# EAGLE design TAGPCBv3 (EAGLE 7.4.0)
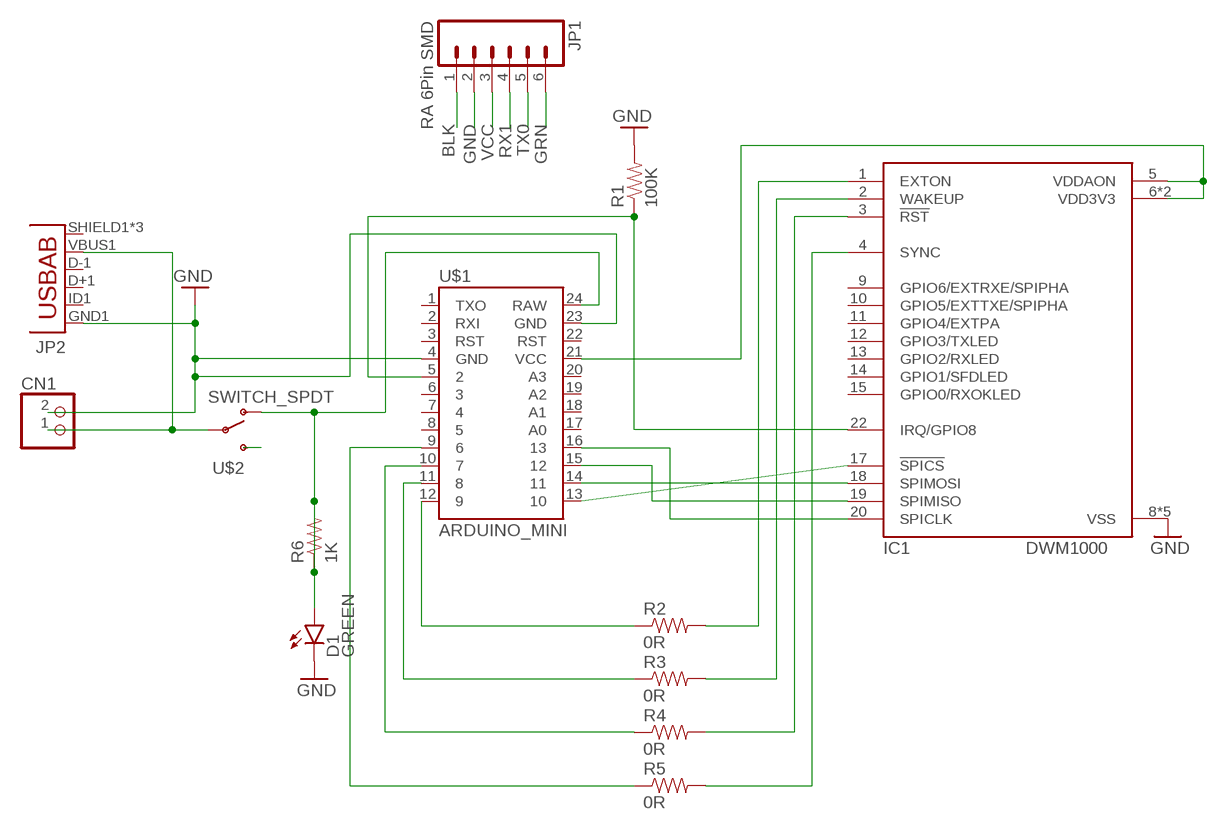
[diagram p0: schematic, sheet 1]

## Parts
CN1  JST_2PIN-SMT-RA  [JST-PH-2-SMT-RA]
D1  GREEN  LED-GREEN0603  [LED-0603]
IC1  DWM1000  [DWM1000]
JP1  RA 6Pin SMD  M06SMD  [1X06-SMD]
JP2  USB-ABCONN-11794  [USB-AB-MICRO-SMD_V03]
R1  100K  RESISTORAXIAL-0.3  [AXIAL-0.3]
R2  0R  RESISTOR1206  [1206]
R3  0R  RESISTOR1206  [1206]
R4  0R  RESISTOR1206  [1206]
R5  0R  RESISTOR1206  [1206]
R6  1K  RESISTOR1206  [1206]
U$1  ARDUINO_MINI  [ARDUINO_MINI]
U$2  SWITCH_SPDT  [KPS-1290]

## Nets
BLK: JP1.1
GND: CN1.2 D1.C IC1.8(VSS) IC1.16(VSS) IC1.21(VSS) IC1.23(VSS) IC1.24(VSS) JP1.2 JP2.GND1(GND) R1.P$2 U$1.4(GND) U$1.23(GND)
GRN: JP1.6
N$1: IC1.17(!SPICS) U$1.13
N$2: IC1.22(IRQ/GPIO8) R1.P$1 U$1.5
N$3: IC1.18(SPIMOSI) U$1.14
N$4: IC1.19(SPIMISO) U$1.15
N$5: IC1.20(SPICLK) U$1.16
N$6: D1.A R6.1 R6.2 U$1.24(RAW) U$2.O
N$7: CN1.1 JP2.VBUS1(VBUS) U$2.P
N$8: IC1.5(VDDAON) IC1.6(VDD3V3) IC1.7(VDD3V3) U$1.21(VCC)
N$9: R2.1 U$1.12
N$10: IC1.1(EXTON) R2.2
N$11: R3.1 U$1.11
N$12: IC1.2(WAKEUP) R3.2
N$13: IC1.3(!RST) R4.2
N$14: R4.1 U$1.10
N$15: R5.1 U$1.9
N$16: IC1.4(SYNC) R5.2
N$17: U$2.S
RX1: JP1.4
TX0: JP1.5
VCC: JP1.3
Unconnected: IC1.9(GPIO6/EXTRXE/SPIPHA) IC1.10(GPIO5/EXTTXE/SPIPHA) IC1.11(GPIO4/EXTPA) IC1.12(GPIO3/TXLED) IC1.13(GPIO2/RXLED) IC1.14(GPIO1/SFDLED) IC1.15(GPIO0/RXOKLED) JP2.D+1(D+) JP2.D-1(D-) JP2.ID1(USBID) JP2.SHIELD1(SHIELD) JP2.SHIELD2(SHIELD) JP2.SHIELD3(SHIELD) U$1.1(TXO) U$1.2(RXI) U$1.3(RST) U$1.6 U$1.7 U$1.8 U$1.17(A0) U$1.18(A1) U$1.19(A2) U$1.20(A3) U$1.22(RST)

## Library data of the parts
CN1 = adafruit:JST_2PIN: JST 2-Pin Connectors of various flavors
D1 = SparkFun-LED:LED-GREEN: Various green LEDs; PROD_ID: DIO-00821
IC1 = decawave:DWM1000
JP1 = SparkFun-Connectors:M06: Header 6 Standard 6-pin 0.1" header. Use with straight break away headers (SKU : PRT-00116), right angle break away headers (PRT-00553), swiss pins (PRT-00743), machine pins (PRT-00117), and female headers (PRT-00115). Molex polarized connector foot print use with SKU : PRT-08094 with associated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; PROD_ID: CONN-08971
JP2 = SparkFun-Connectors:USB-AB: This is a USB AB connector that is compatible with USB OTG. i.e. this connector can serve as a host or device; PROD_ID: CONN-11794
R1-R6 = SparkFun-Resistors:RESISTOR: Resistor
U$1 = SparkFun-Boards:ARDUINO_MINI: Arduino Pro Mini footprint
U$2 = SparkFun-Electromechanical:SWITCH_SPDT: SWCH-10651 Side-actuated SPDT slide switch, as used on the Arduino Pro; PROD_ID: SWCH-10651

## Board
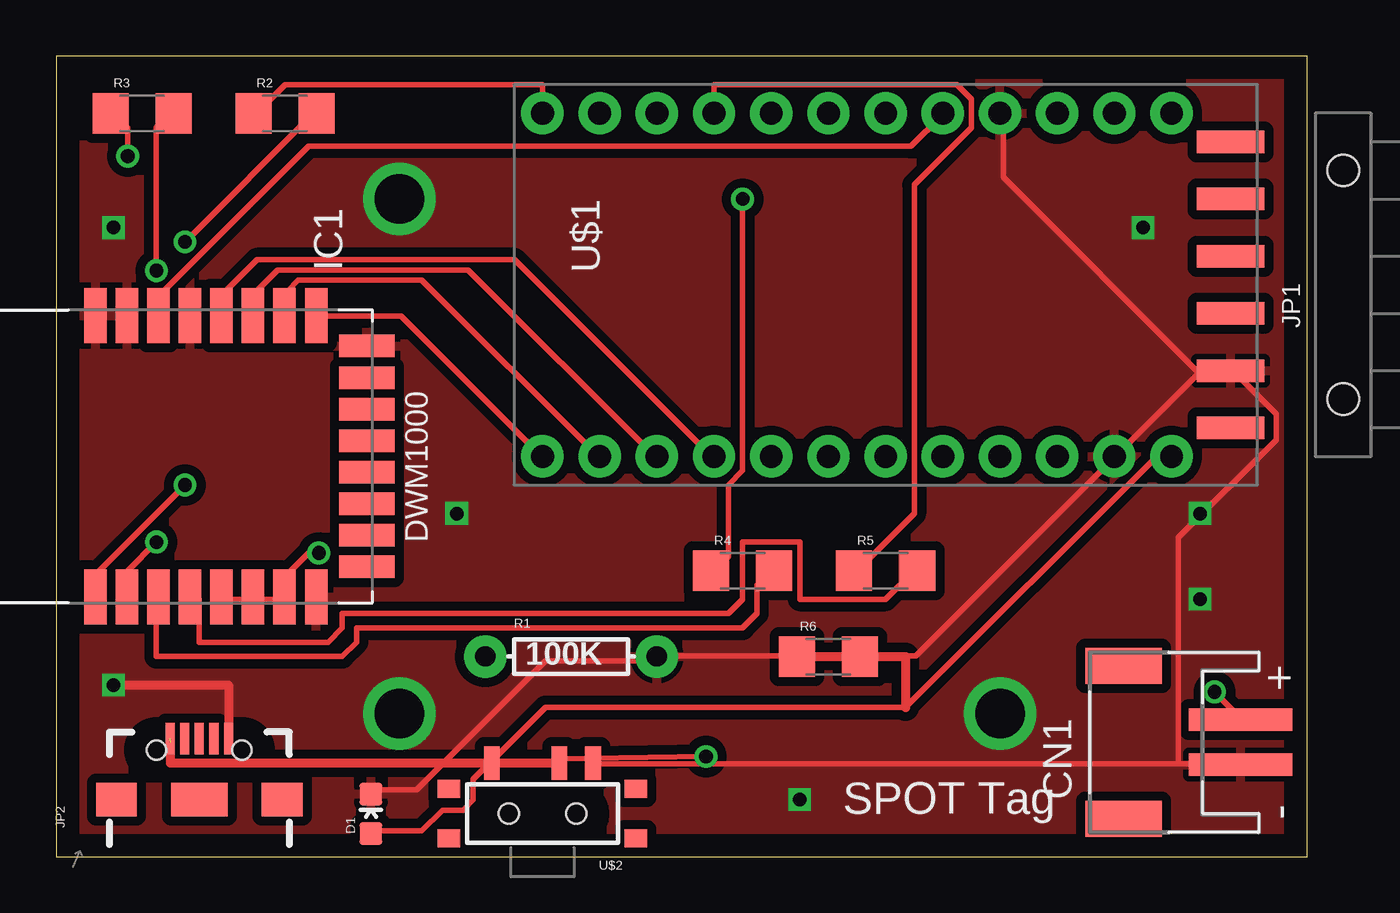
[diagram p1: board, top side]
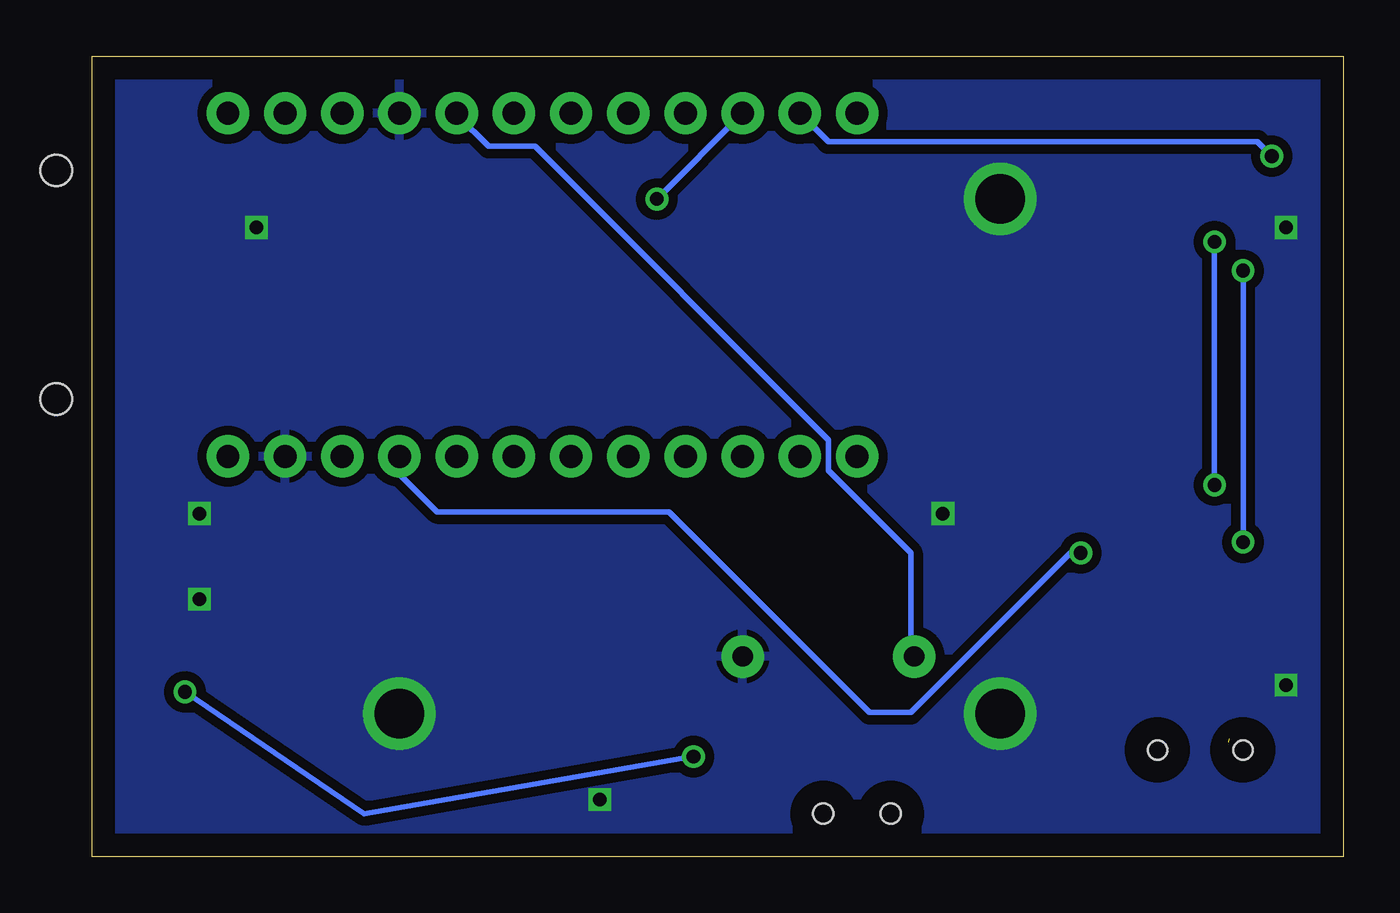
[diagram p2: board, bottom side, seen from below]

Size 55.55 x 35.55 mm. Coordinates in mm from the lower left corner, seen from the top.
Outline: 0,0 55.55,0 55.55,35.55 0,35.55 0,0
Copper layers (1*16): Top 0.035mm / dielectric 1.5mm / Bottom 0.035mm
Design rules "default *": minimum track width 10mil, minimum drill 24mil, track to track 8mil, track to pad 8mil, pad to pad 8mil, via to via 8mil, smd to smd 8mil, copper to edge 40mil, drill to drill 8mil, minimum pad ring 10mil, minimum via ring 8mil, stop-mask expansion 4mil, vias tented up to drill 0mil, thermal gap 10mil

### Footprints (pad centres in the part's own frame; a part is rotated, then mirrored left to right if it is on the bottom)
JST-PH-2-SMT-RA = smd 1 x 4.6: 1 1,-3.7; 2 -1,-3.7 | smd 1.6 x 3.4: NC1 -3.4,1.5; NC2 3.4,1.5
LED-0603 = smd 1 x 1: A 0,-0.877; C 0,0.877
DWM1000 = smd 2.45 x 1: 1 -6.25,0.8; 2 -6.25,-0.6; 3 -6.25,-2; 4 -6.25,-3.4; 5 -6.25,-4.8; 6 -6.25,-6.2; 7 -6.25,-7.6; 8 -6.25,-9; 17 6.25,-9; 18 6.25,-7.6; 19 6.25,-6.2; 20 6.25,-4.8; 21 6.25,-3.4; 22 6.25,-2; 23 6.25,-0.6; 24 6.25,0.8 | smd 1 x 2.45: 9 -4.9,-11.25; 10 -3.5,-11.25; 11 -2.1,-11.25; 12 -0.7,-11.25; 13 0.7,-11.25; 14 2.1,-11.25; 15 3.5,-11.25; 16 4.9,-11.25
1X06-SMD = smd 1 x 3: 1 -6.35,5; 2 -3.81,5; 3 -1.27,5; 4 1.27,5; 5 3.81,5; 6 6.35,5 | hole 1.4: -5.08,0; 5.08,0
USB-AB-MICRO-SMD_V03 = smd 1.4 x 0.4: D+1 2.7,0; D-1 2.7,0.65; GND1 2.7,-1.3; ID1 2.7,-0.65; VBUS1 2.7,1.3 | smd 1.5 x 1.8: SHIELD1 0,3.68; SHIELD3 0,-3.68 | smd 1.5 x 2.5: SHIELD2 0,0 | hole 0.85: 2.2,1.9; 2.2,-1.9
AXIAL-0.3 = drill 0.9 pad 1.88: P$1 -3.81,0; P$2 3.81,0
1206 = smd 1.6 x 1.8: 1 -1.4,0; 2 1.4,0
ARDUINO_MINI = drill 1.016 pad 1.88: 1 -7.62,12.7; 2 -7.62,10.16; 3 -7.62,7.62; 4 -7.62,5.08; 5 -7.62,2.54; 6 -7.62,0; 7 -7.62,-2.54; 8 -7.62,-5.08; 9 -7.62,-7.62; 10 -7.62,-10.16; 11 -7.62,-12.7; 12 -7.62,-15.24; 13 7.62,-15.24; 14 7.62,-12.7; 15 7.62,-10.16; 16 7.62,-7.62; 17 7.62,-5.08; 18 7.62,-2.54; 19 7.62,0; 20 7.62,2.54; 21 7.62,5.08; 22 7.62,7.62; 23 7.62,10.16; 24 7.62,12.7
KPS-1290 = smd 0.7 x 1.5: O -2.25,2.25; P 0.75,2.25; S 2.25,2.25 | smd 1 x 0.8: P$1 -4.15,1.1; P$2 -4.15,-1.1; P$3 4.15,-1.1; P$4 4.15,1.1 | hole 0.9: -1.5,0; 1.5,0

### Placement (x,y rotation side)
CN1  48.9,5.08 90 top
D1  13.97,1.91 0 top
IC1  2.54,17.78 90 top
JP1  57.15,25.4 90 top
JP2  6.35,2.54 90 top
R1  22.86,8.89 0 top
R2  10.16,33.02 0 top
R3  3.81,33.02 0 top
R4  30.48,12.7 0 top
R5  36.83,12.7 0 top
R6  34.29,8.89 0 top
U$1  36.83,25.4 270 top
U$2  21.59,1.91 0 top

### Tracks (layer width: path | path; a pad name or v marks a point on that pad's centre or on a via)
GND  (via drill 0.6, 2.2, 2.2 pad 3.17)
  Top 0.254: 49.84,4.12 52.58,4.12 CN1.2 | 49.84,4.12 24,4.12 | D1.C 14.17,2.97 16,2.97 21.72,8.69 26.52,8.69 R1.P$2 26.75,8.91 38.18,8.91 46.86,17.6 U$1.23 47.09,17.83 50.75,21.49 | 50.75,21.49 52.12,21.49 JP1.2 | 50.75,21.49 42.06,30.18 42.06,32.92 U$1.4 | 50.75,21.49 JP1.2 | 49.84,4.12 49.84,14.17 54.18,18.52 54.18,19.66 52.35,21.49 JP1.2
  Top 0.406: v2.54,7.62 7.65,7.62 JP2.GND1
  other vias: 2.54,27.94 17.78,15.24 15.24,29.21 33.02,2.54 41.91,6.35 48.26,27.94 15.24,6.35 50.8,11.43 50.8,15.24
  pour Bottom (isolate 0.406): 0,0 0,35.56 55.88,35.56 55.88,0
  pour Top (isolate 0.406): 0,0 0,35.56 55.88,35.56 55.88,34.29 55.88,0
N$1
  Top 0.254: IC1.17 11.66,24 15.32,24 21.49,17.83 U$1.13
N$2
  Top 0.254: IC1.22 4.57,24.23 4.57,24.92 11.2,31.55 37.95,31.55 39.32,32.92 U$1.5
  Bottom 0.254: R1.P$1 19.2,8.91 19.2,13.49 22.86,17.14 22.86,18.52 35.89,31.55 37.95,31.55 39.32,32.92 U$1.5
N$3
  Top 0.254: IC1.18 10.29,24.23 10.29,25.15 10.74,25.6 16.23,25.6 24,17.83 U$1.14
N$4
  Top 0.254: IC1.19 8.91,24.23 8.91,25.15 9.83,26.06 18.29,26.06 26.52,17.83 U$1.15
N$5
  Top 0.254: IC1.20 7.54,24.23 7.54,25.15 8.91,26.52 20.34,26.52 29.03,17.83 U$1.16
N$6
  Top 0.254: D1.A 14.17,1.14 16.23,1.14 17.14,2.06 18.06,2.06 18.52,2.52 18.52,3.43 19.2,4.12 U$2.O 19.43,4.34 21.72,6.63 37.72,6.63 48.69,17.6 49.38,17.6 U$1.24
  Top 0.406: R6.1 R6.2 37.72,8.89 37.72,6.63
N$7  (via drill 0.61)  (1 unrouted)
  Top 0.254: v28.85,4.45 22.4,4.34 U$2.P | v51.44,7.32 52.58,6.17 CN1.1
  Top 0.406: U$2.P 5.08,4.16 5.08,5.08
  Bottom 0.254: v28.85,4.45 43.48,1.91 v51.44,7.32
N$8  (via drill 0.61)
  Top 0.254: IC1.5 7.54,11.43 8.69,11.43 IC1.6 8.91,11.43 10.06,11.43 IC1.7 10.29,11.66 10.29,12.57 11.2,13.49 v11.66,13.49
  Bottom 0.254: v11.66,13.49 12.12,13.49 19.2,6.4 21.03,6.4 29.95,15.32 40.23,15.32 41.83,16.92 41.83,17.6 U$1.21
N$9
  Top 0.254: U$1.12 21.59,34.29 10.16,34.29 8.89,33.02 R2.1
N$10  (via drill 0.61)
  Top 0.254: v5.71,27.3 11.43,33.02 R2.2 | v5.71,16.51 1.91,12.7 1.91,12.06 IC1.1
  Bottom 0.254: v5.71,16.51 v5.71,27.3
N$11  (via drill 0.61)
  Top 0.254: v3.17,31.11 3.17,32.38 2.54,33.02 R3.1
  Bottom 0.254: v3.17,31.11 3.81,31.75 22.86,31.75 U$1.11
N$12  (via drill 0.61)
  Top 0.254: v4.45,26.04 4.45,32.38 5.08,33.02 R3.2 | v4.45,13.97 3.17,12.7 3.17,12.06 IC1.2
  Bottom 0.254: v4.45,13.97 v4.45,26.04
N$13
  Top 0.254: R4.2 31.75,12.7 31.11,12.06 31.11,10.79 30.48,10.16 13.34,10.16 13.34,9.53 12.7,8.89 4.45,8.89 4.45,11.43 IC1.3
N$14  (via drill 0.61)
  Top 0.254: v30.48,29.21 30.48,17.14 29.84,16.51 29.84,13.34 29.21,12.7 R4.1
  Bottom 0.254: U$1.10 v30.48,29.21
N$15
  Top 0.254: U$1.9 29.21,34.29 40.01,34.29 40.64,33.66 40.64,32.38 38.1,29.84 38.1,15.24 35.56,12.7 R5.1
N$16
  Top 0.254: R5.2 38.1,12.7 36.83,11.43 33.02,11.43 33.02,13.97 30.48,13.97 30.48,11.43 29.84,10.79 12.7,10.79 12.7,10.16 12.06,9.53 6.35,9.53 6.35,11.43 IC1.4

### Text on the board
tSilk: DWM1000 | SPOT Tag

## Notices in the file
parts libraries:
SparkFun-Boards: Licensing: Creative Commons ShareAlike 4.0 International - https://creativecommons.org/licenses/by-sa/4.0
